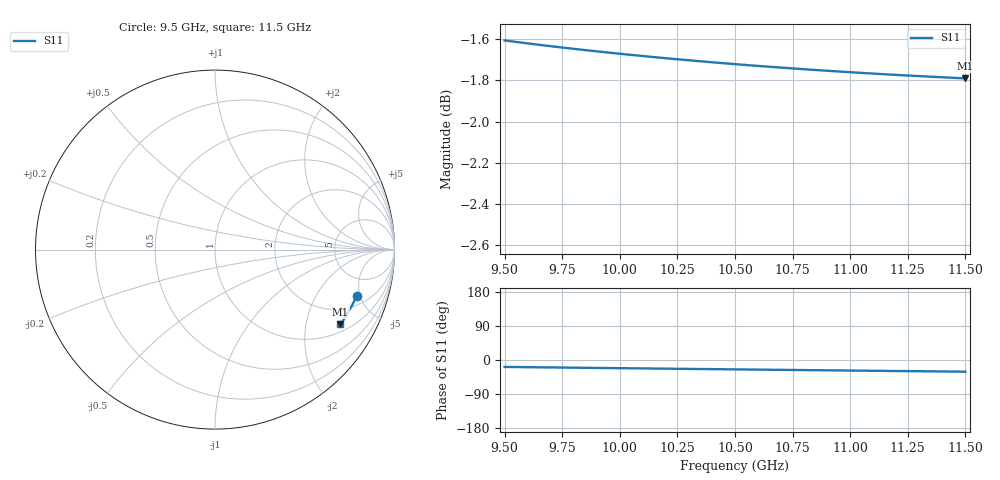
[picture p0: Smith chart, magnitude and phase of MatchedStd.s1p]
# GHZ S RI R 50
!Output file by EM3DS 6.2.15 Beta
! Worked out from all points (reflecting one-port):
!   101 points, 9.5 GHz to 11.5 GHz, reference 50 ohm
!   lowest |S11| = -1.8 dB at 11.5 GHz (marker M1), VSWR 9.74, Z = 63.9 - j158 ohm
!   phase of S11 starts at -18 deg and turns -13 deg over the sweep
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9.5  0.7894 -0.2604
9.56  0.7867 -0.2658
9.62  0.7841 -0.271
9.7  0.7806 -0.278
9.76  0.7779 -0.2832
9.84  0.7744 -0.29
9.88  0.7726 -0.2934
9.92  0.7708 -0.2967
10  0.7672 -0.3034
10.08  0.7637 -0.31
10.12  0.7619 -0.3133
10.16  0.7601 -0.3166
10.26  0.7556 -0.3247
10.32  0.7529 -0.3295
10.38  0.7502 -0.3342
10.46  0.7466 -0.3405
10.52  0.7439 -0.3452
10.64  0.7385 -0.3545
10.76  0.733 -0.3636
10.86  0.7285 -0.3711
10.94  0.7248 -0.377
11.02  0.7211 -0.3829
11.12  0.7165 -0.3901
11.2  0.7128 -0.3959
11.26  0.71 -0.4001
11.3  0.7082 -0.403
11.38  0.7045 -0.4086
11.5  0.6989 -0.4169
